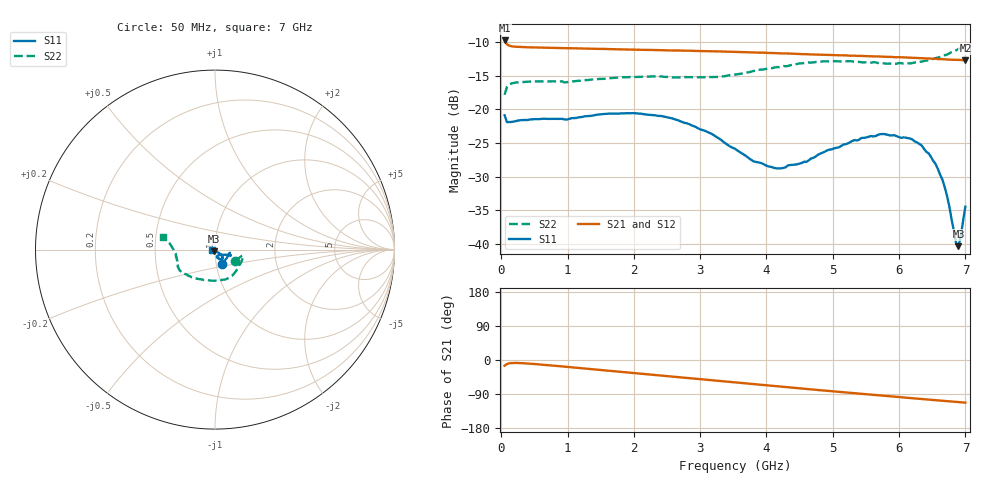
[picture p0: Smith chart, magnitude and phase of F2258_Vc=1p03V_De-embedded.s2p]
! Integrated Device Technology
! Corporate Headquarters
! 6024 Silver Creek Valley Road
! San Jose, CA 95138  USA
! Phone:  1-408-284-8200
! Toll Free:  1-800-223-1366
! Webpage:  http://www.idt.com/
! Timing and RF Division
! 515 Groton Road, Suite 102
! Westford, MA 01886-6024
! Device:  F2258
! Description: Voltage Variable RF Attenuator
! Frequency:  50.0 -  6000.00 MHz
! Package:  3x3 mm Thin QFN Plastic Package: 16 pin
! Ports:  2 RF, 2 DC
!  Pin  1  = NC
!  Pin  2  = NC
!  Pin  3  = RF2  = Port 2
!  Pin  4  = GND
!  Pin  5  = Vdd
!  Pin  6  = NC
!  Pin  7  = VCTRL
!  Pin  8  = NC
!  Pin  9  = GND
!  Pin 10  = RF1  = Port 1
!  Pin 11  = NC
!  Pin 12  = NC
!  Pin 13  = NC
!  Pin 14  = NC
!  Pin 15  = NC
!  Pin 16  = NC
! Vcntrl:  1.030 Volts
! Vdd:  +3.300 Volts
! Current:  1.158 mA
! Data:  The device was measured on a the F2258 evaluation board which has
!  individual transmission lines to the RF pins.  Data was collected
!  using a calibrated network analyzer.  The evaluation board was
!  de-embedded using a TRL calibration technique.
!  The reference plane is the edge of the package pin.
! Misc:  SN 10
!  Action Tracker AT0285
! Date Measured:  2014-12-10
! Date:  2016-01-13  MJV
! Note:
!  Integrated Device Technology supplies this data as a sample of measured
!  data at the package pin for this product.  Your particular data for this
!  product may vary.
!  Data was taken at 25 degrees C.
!  Integrated Device Technology reserves the right to change this data at anytime.
!Freq_(GHz)  S11M_(dB)  S11P_(deg)  S21M_(dB)  S21P_(deg)  S12M_(dB)  S12P_(deg)  S22M_(dB)  S22P_(deg)
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# GHz S dB R 50
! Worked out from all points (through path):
!   201 points, 50 MHz to 7 GHz, reference 50 ohm
!   highest |S21| = -9.74 dB at 50 MHz (marker M1); lowest = -12.7 dB at 7 GHz (marker M2)
!   group delay of S21, straight-line fit = 43.7 ps
!   lowest |S11| = -40.3 dB at 6.896 GHz (marker M3), VSWR 1.02, Z = 49.5 - j0.835 ohm
!   |S11| at or under -10 dB: start of sweep to end of sweep
!   |S22| runs from -17.8 to -10.5 dB; largest |S21 - S12| = 0.0011
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0.05  -20.85 -66.2  -9.74 -15.1  -9.75 -15.1  -17.81 -29.4
0.08475  -21.87 -38.3  -10.33 -10.6  -10.33 -10.6  -16.66 -16.1
0.189  -21.80 -17.3  -10.65 -7.8  -10.66 -7.8  -16.05 -11.7
1.2315  -21.08 -18.7  -10.94 -22.0  -10.94 -22.0  -15.66 -40.6
1.9265  -20.55 -20.1  -11.09 -33.0  -11.10 -33.0  -15.18 -58.9
2.37825  -20.95 -20.5  -11.19 -40.3  -11.17 -40.3  -15.09 -71.2
3.07325  -23.17 -24.8  -11.32 -51.6  -11.33 -51.6  -15.20 -94.8
3.525  -25.83 -34.6  -11.42 -59.1  -11.44 -59.1  -14.81 -113.1
3.803  -27.70 -47.6  -11.52 -63.7  -11.54 -63.6  -14.28 -123.6
4.1505  -28.75 -62.8  -11.63 -69.3  -11.63 -69.2  -13.71 -134.1
4.7065  -27.18 -74.1  -11.82 -78.0  -11.81 -78.0  -13.00 -146.5
5.43625  -24.22 -61.2  -12.04 -89.2  -12.05 -89.2  -12.99 -157.6
5.85325  -23.84 -50.0  -12.19 -95.5  -12.17 -95.6  -13.17 -166.1
6.20075  -24.47 -44.0  -12.32 -100.9  -12.31 -100.9  -13.10 -174.6
6.33975  -25.34 -41.1  -12.37 -103.0  -12.38 -103.0  -12.87 -178.2
6.54825  -28.06 -40.1  -12.46 -106.1  -12.48 -106.1  -12.38 176.6
6.68725  -31.52 -43.2  -12.55 -108.0  -12.56 -108.0  -11.94 173.1
6.75675  -34.35 -49.5  -12.59 -109.1  -12.61 -109.0  -11.66 171.1
6.861  -39.96 -88.7  -12.61 -110.6  -12.63 -110.5  -11.20 169.2
6.89575  -40.31 -119.1  -12.63 -111.1  -12.66 -111.0  -11.01 168.5
6.9305  -38.85 -138.0  -12.64 -111.5  -12.66 -111.5  -10.89 168.1
7  -34.43 -170.5  -12.68 -112.5  -12.71 -112.5  -10.52 166.5
